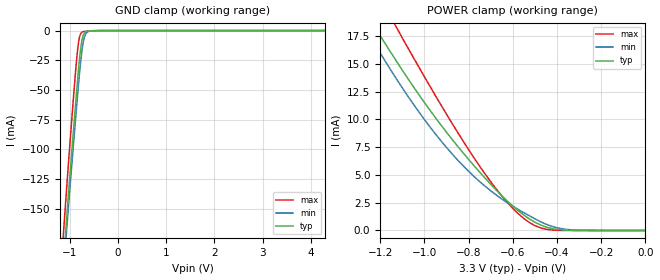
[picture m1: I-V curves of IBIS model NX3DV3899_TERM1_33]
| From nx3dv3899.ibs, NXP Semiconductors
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| Remark: If your software does not support the Model Selector
|   Please comment out the lines of the Model Selector, which
|   contain the name of the Model, except the one you want to use.
|   Model NX3DV3899_TERM1_33
[Model]   NX3DV3899_TERM1_33
Model_type   Terminator
C_comp   32.2940pF   29.6500pF   35.6150pF
| ON capacitance of switch
|Ambient temperature:   25   85   -40
[Temperature Range]   30   90   -35
[Voltage Range]   3.3   3.0   3.6
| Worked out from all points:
|   GND clamp passes 1 mA (typ) near -0.67 V on its own axis
|   POWER clamp passes 1 mA (typ) near -0.52 V on its own axis
|Process Range   nominal   slow   fast
[GND_clamp]
|   voltage   I(typ)   I(min)   I(max)
-4.3V     -2.187A    -2.175A    -2.181A
-1.13V    -194.8mA   -203.5mA   -169.8mA
-1.078V   -165.4mA   -174.8mA   -139.8mA
-1.061V   -155.9mA   -165.5mA   -130mA
-921.7mV  -83.15mA   -94.91mA   -55.3mA
-852.2mV  -48.16mA   -60.83mA   -21.84mA
-800mV    -24.46mA   -36.63mA   -5.762mA
-747.8mV  -8.11mA    -16.82mA   -1.331mA
-713mV    -3.133mA   -8.174mA   -812.2uA
-678.3mV  -1.287mA   -3.511mA   -619.9uA
-539.1mV  -226.2uA   -304.6uA   -204uA
4.3V      0A         0A         0A
[POWER_clamp]
|   voltage   I(typ)   I(min)   I(max)
-4.3V     373.4mA    303.3mA    504.1mA
-1.275V   19.96mA    18.5mA     24.04mA
-1.25V    19.14mA    17.65mA    23.02mA
-1.2V     17.53mA    15.98mA    21.04mA
-1.125V   15.19mA    13.6mA     18.23mA
-975mV    10.83mA    9.328mA    12.98mA
-825mV    6.989mA    5.826mA    8.054mA
-675mV    3.638mA    3.195mA    3.735mA
-550mV    1.382mA    1.6mA      1.075mA
-475mV    498.7uA    791.8uA    237.2uA
-375mV    45.67uA    146.3uA    5.864uA
0V        88.86pA    1.589nA    634.8fA
